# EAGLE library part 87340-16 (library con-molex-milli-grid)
RECEPTACAL
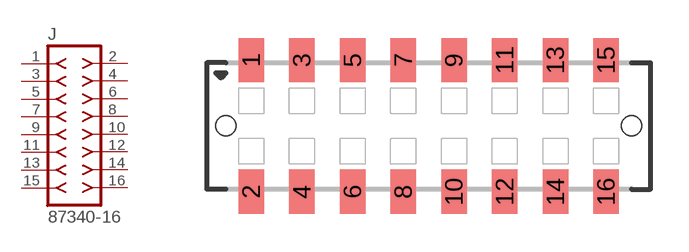
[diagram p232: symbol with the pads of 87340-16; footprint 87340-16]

Designator prefix J

## 87340-16  [87340-16]
1  1  pas
2  2  pas
3  3  pas
4  4  pas
5  5  pas
6  6  pas
7  7  pas
8  8  pas
9  9  pas
10  10  pas
11  11  pas
12  12  pas
13  13  pas
14  14  pas
15  15  pas
16  16  pas

## Footprint 87340-16 (pad centres in mm)
RECEPTACAL SMD Dual Row, Vertical, Low Profile
smd 1 x 1.75: 1 -7,2.6; 2 -7,-2.6; 3 -5,2.6; 4 -5,-2.6; 5 -3,2.6; 6 -3,-2.6; 7 -1,2.6; 8 -1,-2.6; 9 1,2.6; 10 1,-2.6; 11 3,2.6; 12 3,-2.6; 13 5,2.6; 14 5,-2.6; 15 7,2.6; 16 7,-2.6
hole 0.8 at -8,0
hole 0.8 at 8,0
